DATA_BLOCK DB219
TITLE =

AUTHOR:nb
FAMILY:nb
NAME:nb
VERSION:00.01


  STRUCT
   Data : ARRAY  [1 .. 8 ] OF BYTE
   CANopenError : DWORD
   RetVal : WORD
  END_STRUCT

BEGIN
       Data[1]:=B#16#00
       Data[2]:=B#16#00
       Data[3]:=B#16#00
       Data[4]:=B#16#00
       Data[5]:=B#16#00
       Data[6]:=B#16#00
       Data[7]:=B#16#00
       Data[8]:=B#16#00
       CANopenError:=DW#16#00000000
       RetVal:=W#16#0000

END_DATA_BLOCK
